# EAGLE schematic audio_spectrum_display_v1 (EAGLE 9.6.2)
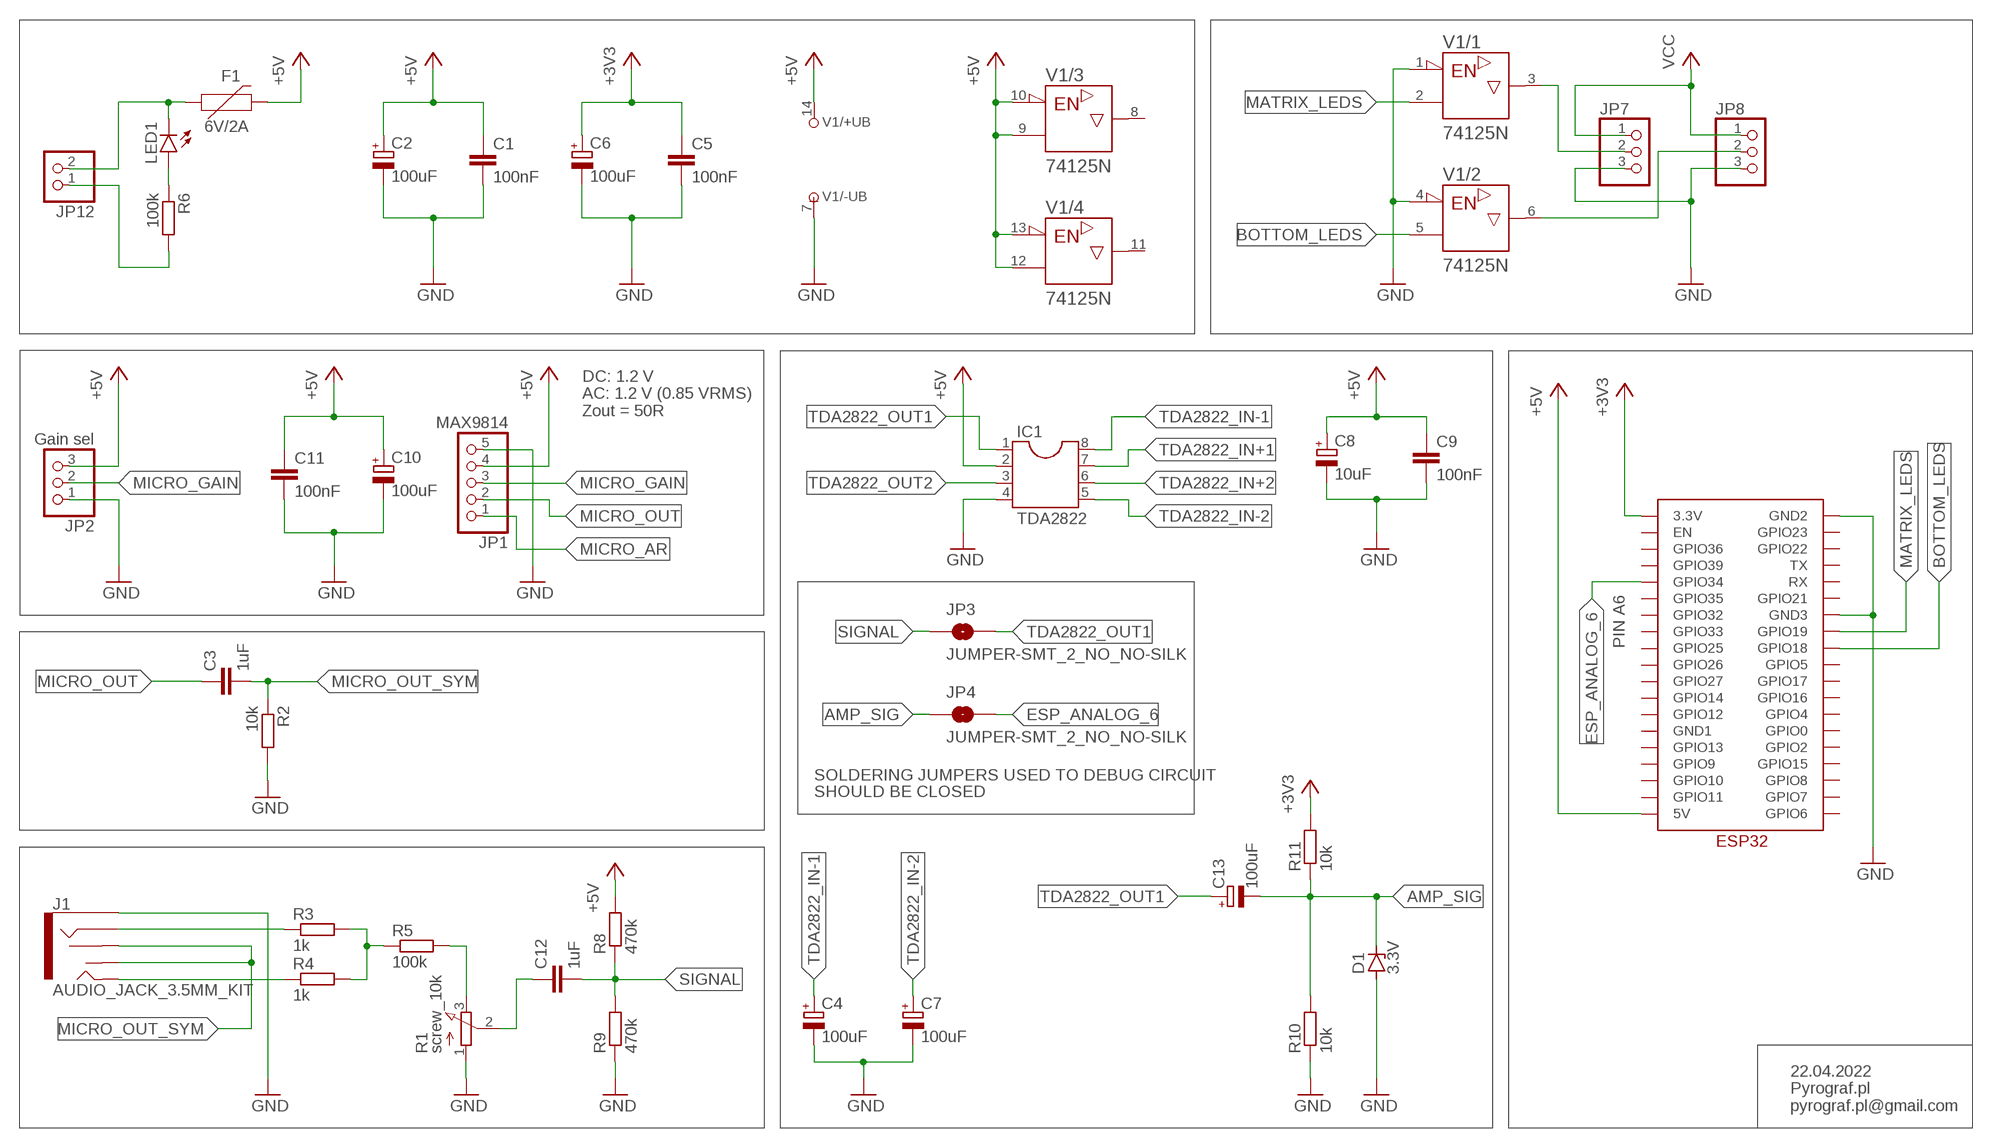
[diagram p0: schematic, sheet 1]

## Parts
C1  100nF  C-EU025-025X050  [C025-025X050]
C2  100uF  CPOL-EUE2.5-7  [E2,5-7]
C3  1uF  C-EU025-025X050  [C025-025X050]
C4  100uF  CPOL-EUE2.5-7  [E2,5-7]
C5  100nF  C-EU025-025X050  [C025-025X050]
C6  100uF  CPOL-EUE2.5-7  [E2,5-7]
C7  100uF  CPOL-EUE2.5-7  [E2,5-7]
C8  10uF  CPOL-EUE2.5-7  [E2,5-7]
C9  100nF  C-EU025-025X050  [C025-025X050]
C10  100uF  CPOL-EUE2.5-7  [E2,5-7]
C11  100nF  C-EU025-025X050  [C025-025X050]
C12  1uF  C-EU025-025X050  [C025-025X050]
C13  100uF  CPOL-EUE2.5-7  [E2,5-7]
D1  3.3V  ZENER-DIODEDO34-7  [DO34Z7]
F1  6V/2A  PPTC_6V2A  [1210]
IC1  TDA2822  DIL8  [DIL08]
J1  AUDIO_JACK_3.5MM_KIT  [AUDIO-JACK-KIT]
JP1  MAX9814  PINHD-1X5/90  [1X05/90]
JP2  Gain sel  PINHD-1X3/90  [1X03/90]
JP3  JUMPER-SMT_2_NO_NO-SILK  [SMT-JUMPER_2_NO_NO-SILK]
JP4  JUMPER-SMT_2_NO_NO-SILK  [SMT-JUMPER_2_NO_NO-SILK]
JP7  PINHD-1X3  [1X03]
JP8  PINHD-1X3  [1X03]
JP12  PINHD-1X2  [1X02]
LED1  LED5MM  [LED5MM]
R1  screw_10k  3RP/1610N  [3RP/1610N]
R2  10k  R-EU_0207/7  [0207/7]
R3  1k  R-EU_0207/7  [0207/7]
R4  1k  R-EU_0207/7  [0207/7]
R5  100k  R-EU_0207/7  [0207/7]
R6  100k  R-EU_0207/7  [0207/7]
R8  470k  R-EU_0207/7  [0207/7]
R9  470k  R-EU_0207/7  [0207/7]
R10  10k  R-EU_0207/7  [0207/7]
R11  10k  R-EU_0207/7  [0207/7]
U$2  ESP32  [ESP32]
V1  74125N  [DIL14]

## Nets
+3V3: C5.1 C6.+ R11.2 U$2.3.3V
+5V: C1.1 C2.+ C8.+ C9.1 C10.+ C11.1 F1.2 IC1.2 JP1.4 JP2.3 R8.2 U$2.5V V1.9(/3:A) V1.10(/3:!G) V1.12(/4:A) V1.13(/4:!G) V1.14(/+UB:+UB)
AMP_SIG: C13.- D1.C JP4.1 R10.2 R11.1
BOTTOM_LEDS: U$2.GPIO18 V1.5(/2:A)
ESP_ANALOG_6: JP4.2 U$2.GPIO34
GND: C1.2 C2.- C4.- C5.2 C6.- C7.- C8.- C9.2 C10.- C11.2 D1.A IC1.4 J1.SLEEVE JP1.5 JP2.1 JP7.3 JP8.3 R1.1(A) R2.2 R9.1 R10.1 U$2.GND2 U$2.GND3 V1.1(/1:!G) V1.4(/2:!G) V1.7(/-UB:-UB)
MATRIX_LEDS: U$2.GPIO19 V1.2(/1:A)
MICRO_AR: JP1.1
MICRO_GAIN: JP1.3 JP2.2
MICRO_OUT: C3.1 JP1.2
MICRO_OUT_SYM: C3.2 J1.RSH J1.TSH R2.1
N$1: J1.TIP R4.1
N$2: F1.1 JP12.2 LED1.K(C)
N$3: C12.1 R1.2(S)
N$4: R1.3(E) R5.2
N$5: J1.RING R3.1
N$6: JP8.2 V1.6(/2:Y)
N$7: R3.2 R4.2 R5.1
N$8: JP7.2 V1.3(/1:Y)
N$9: JP12.1 R6.2
N$10: LED1.A R6.1
SIGNAL: C12.2 JP3.1 R8.1 R9.2
TDA2822_IN+1: IC1.7
TDA2822_IN+2: IC1.6
TDA2822_IN-1: C4.+ IC1.8
TDA2822_IN-2: C7.+ IC1.5
TDA2822_OUT1: C13.+ IC1.1 JP3.2
TDA2822_OUT2: IC1.3
VCC: JP7.1 JP8.1
Unconnected: U$2.EN U$2.GND1 U$2.GPIO0 U$2.GPIO2 U$2.GPIO4 U$2.GPIO5 U$2.GPIO6 U$2.GPIO7 U$2.GPIO8 U$2.GPIO9 U$2.GPIO10 U$2.GPIO11 U$2.GPIO12 U$2.GPIO13 U$2.GPIO14 U$2.GPIO15 U$2.GPIO16 U$2.GPIO17 U$2.GPIO21 U$2.GPIO22 U$2.GPIO23 U$2.GPIO25 U$2.GPIO26 U$2.GPIO27 U$2.GPIO32 U$2.GPIO33 U$2.GPIO35 U$2.GPIO36 U$2.GPIO39 U$2.RX U$2.TX V1.8(/3:Y) V1.11(/4:Y)

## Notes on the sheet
- DC: 1.2 V
  AC: 1.2 V (0.85 VRMS)
  Zout = 50R
- PIN A6
- SOLDERING JUMPERS USED TO DEBUG CIRCUIT
- SHOULD BE CLOSED
- 22.04.2022
  Pyrograf.pl
  pyrograf.pl@gmail.com

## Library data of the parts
C1 C3 C5 C9 C11 C12 = rcl:C-EU: CAPACITOR, European symbol; SPICEPREFIX: C
C2 C4 C6-C8 C10 C13 = rcl:CPOL-EU: POLARIZED CAPACITOR, European symbol; SPICEPREFIX: C
D1 = diode:ZENER-DIODE: Z-Diode
F1 = SparkFun-Fuses:PPTC: Resettable Fuse PPTC; PROD_ID: RES-14313
IC1 = ic-package:DIL8: Dual In Line / Socket
J1 = SparkFun-Connectors:AUDIO_JACK_3.5MM: Audio Jack 3.5mm variants of PTH and SMT stereo audio jack with bypass switches. SparkFun Products: SparkFun SparkPunk Sound Kit - PTH MP3 Trigger -3.5mm SMD SparkFun PicoBoard- 2.5mm SMD; PROD_ID: CONN-08774; SF_ID: PRT-08032
JP1 = pinhead:PINHD-1X5: PIN HEADER
JP2 JP7 JP8 = pinhead:PINHD-1X3: PIN HEADER
JP3 JP4 = SparkFun-Jumpers:JUMPER-SMT_2_NO: Normally open jumper
JP12 = pinhead:PINHD-1X2: PIN HEADER
LED1 = led:LED: LED
R1 = pot:3RP/1610N: 16mm Potentiometer one level Source: http://www.alphapotentiometers.net/html/16mm_pot_2.html
R2-R6 R8-R11 = rcl:R-EU_: RESISTOR, European symbol; SPICEPREFIX: R
U$2 = ESP32:ESP32
V1 = 74ttl-din:74*125: Quad bus BUFFER, 3-state

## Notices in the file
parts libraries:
SparkFun-Fuses: Licensing: Creative Commons ShareAlike 4.0 International - https://creativecommons.org/licenses/by-sa/4.0
